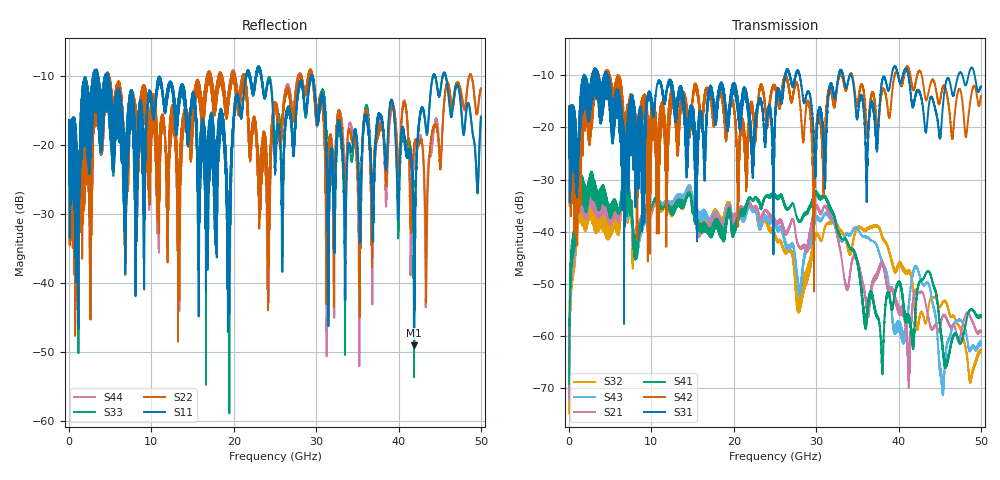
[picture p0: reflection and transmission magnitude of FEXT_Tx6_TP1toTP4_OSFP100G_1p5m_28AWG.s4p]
! Touchstone data
! Created: 27-Feb-2019 by IdEM 12 (12.1.0)
! COMMENTS
!  Created Wed Feb 27 09:43:39 2019
!  64 Port Network Data from SP1.SP block
!  freq  magS1_1  angS1_1  magS1_2  angS1_2  magS1_3  angS1_3  magS1_4  angS1_4
!  magS1_5  angS1_5  magS1_6  angS1_6  magS1_7  angS1_7  magS1_8  angS1_8
!  magS1_9  angS1_9  magS1_10  angS1_10  magS1_11  angS1_11  magS1_12  angS1_12
!  magS1_13  angS1_13  magS1_14  angS1_14  magS1_15  angS1_15  magS1_16  angS1_16
!  magS1_17  angS1_17  magS1_18  angS1_18  magS1_19  angS1_19  magS1_20  angS1_20
!  magS1_21  angS1_21  magS1_22  angS1_22  magS1_23  angS1_23  magS1_24  angS1_24
!  magS1_25  angS1_25  magS1_26  angS1_26  magS1_27  angS1_27  magS1_28  angS1_28
!  magS1_29  angS1_29  magS1_30  angS1_30  magS1_31  angS1_31  magS1_32  angS1_32
!  magS1_33  angS1_33  magS1_34  angS1_34  magS1_35  angS1_35  magS1_36  angS1_36
!  magS1_37  angS1_37  magS1_38  angS1_38  magS1_39  angS1_39  magS1_40  angS1_40
!  magS1_41  angS1_41  magS1_42  angS1_42  magS1_43  angS1_43  magS1_44  angS1_44
!  magS1_45  angS1_45  magS1_46  angS1_46  magS1_47  angS1_47  magS1_48  angS1_48
!  magS1_49  angS1_49  magS1_50  angS1_50  magS1_51  angS1_51  magS1_52  angS1_52
!  magS1_53  angS1_53  magS1_54  angS1_54  magS1_55  angS1_55  magS1_56  angS1_56
!  magS1_57  angS1_57  magS1_58  angS1_58  magS1_59  angS1_59  magS1_60  angS1_60
!  magS1_61  angS1_61  magS1_62  angS1_62  magS1_63  angS1_63  magS1_64  angS1_64
!  magS2_1  angS2_1  magS2_2  angS2_2  magS2_3  angS2_3  magS2_4  angS2_4
!  magS2_5  angS2_5  magS2_6  angS2_6  magS2_7  angS2_7  magS2_8  angS2_8
!  magS2_9  angS2_9  magS2_10  angS2_10  magS2_11  angS2_11  magS2_12  angS2_12
!  magS2_13  angS2_13  magS2_14  angS2_14  magS2_15  angS2_15  magS2_16  angS2_16
!  magS2_17  angS2_17  magS2_18  angS2_18  magS2_19  angS2_19  magS2_20  angS2_20
!  magS2_21  angS2_21  magS2_22  angS2_22  magS2_23  angS2_23  magS2_24  angS2_24
!  magS2_25  angS2_25  magS2_26  angS2_26  magS2_27  angS2_27  magS2_28  angS2_28
!  magS2_29  angS2_29  magS2_30  angS2_30  magS2_31  angS2_31  magS2_32  angS2_32
!  magS2_33  angS2_33  magS2_34  angS2_34  magS2_35  angS2_35  magS2_36  angS2_36
!  magS2_37  angS2_37  magS2_38  angS2_38  magS2_39  angS2_39  magS2_40  angS2_40
!  magS2_41  angS2_41  magS2_42  angS2_42  magS2_43  angS2_43  magS2_44  angS2_44
!  magS2_45  angS2_45  magS2_46  angS2_46  magS2_47  angS2_47  magS2_48  angS2_48
!  magS2_49  angS2_49  magS2_50  angS2_50  magS2_51  angS2_51  magS2_52  angS2_52
!  magS2_53  angS2_53  magS2_54  angS2_54  magS2_55  angS2_55  magS2_56  angS2_56
!  magS2_57  angS2_57  magS2_58  angS2_58  magS2_59  angS2_59  magS2_60  angS2_60
!  magS2_61  angS2_61  magS2_62  angS2_62  magS2_63  angS2_63  magS2_64  angS2_64
!  magS3_1  angS3_1  magS3_2  angS3_2  magS3_3  angS3_3  magS3_4  angS3_4
!  magS3_5  angS3_5  magS3_6  angS3_6  magS3_7  angS3_7  magS3_8  angS3_8
!  magS3_9  angS3_9  magS3_10  angS3_10  magS3_11  angS3_11  magS3_12  angS3_12
!  magS3_13  angS3_13  magS3_14  angS3_14  magS3_15  angS3_15  magS3_16  angS3_16
!  magS3_17  angS3_17  magS3_18  angS3_18  magS3_19  angS3_19  magS3_20  angS3_20
!  magS3_21  angS3_21  magS3_22  angS3_22  magS3_23  angS3_23  magS3_24  angS3_24
!  magS3_25  angS3_25  magS3_26  angS3_26  magS3_27  angS3_27  magS3_28  angS3_28
!  magS3_29  angS3_29  magS3_30  angS3_30  magS3_31  angS3_31  magS3_32  angS3_32
!  magS3_33  angS3_33  magS3_34  angS3_34  magS3_35  angS3_35  magS3_36  angS3_36
!  magS3_37  angS3_37  magS3_38  angS3_38  magS3_39  angS3_39  magS3_40  angS3_40
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# Hz S MA R 50
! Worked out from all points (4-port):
!   5000 points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, 10 MHz to 50 GHz, reference 50 ohm
!   strongest paths, dB at 10 MHz, 12.51 GHz, 25.01 GHz, 37.51 GHz, 50 GHz:
!     S31: -19.6, -12.0, -18.5, -21.3, -12.1
!     S42: -19.6, -15.1, -12.3, -20.3, -14.0
!     S41: -69.3, -36.1, -32.9, -56.7, -56.1
!     S21: -72.0, -35.7, -37.7, -47.4, -59.1
!     S43: -72.2, -34.7, -37.9, -43.4, -61.0
!     S32: -74.9, -35.6, -40.6, -38.9, -63.0
!   lowest |S11| = -49.0 dB at 41.91 GHz (marker M1), VSWR 1.01, Z = 50 - j0.352 ohm
!   |S11| at or under -10 dB: 4.762 GHz to 21.49 GHz (16.73 GHz wide, 127 % of centre); 23.37 GHz to 29.37 GHz (5.999 GHz wide, 22.7 % of centre); 29.57 GHz to 44.19 GHz (14.62 GHz wide, 39.6 % of centre)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
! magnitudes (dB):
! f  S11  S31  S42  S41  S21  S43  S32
! 10 MHz  -19.1  -19.6  -19.6  -69.3  -72.0  -72.2  -74.9
! 1.36 GHz  -19.4  -18.6  -22.5  -30.2  -31.7  -32.0  -33.9
! 6.69 GHz  -30.3  -24.9  -21.6  -29.7  -30.0  -30.0  -30.6
! 19.39 GHz  -32.2  -18.9  -16.7  -36.1  -35.3  -35.1  -34.9
! 29.47 GHz  -9.8  -16.5  -22.7  -34.6  -38.3  -41.3  -44.1
! 41.91 GHz  -49.0  -15.3  -12.6  -58.7  -51.7  -46.9  -52.8
! 50 GHz  -15.9  -12.1  -14.0  -56.1  -59.1  -61.0  -63.0
